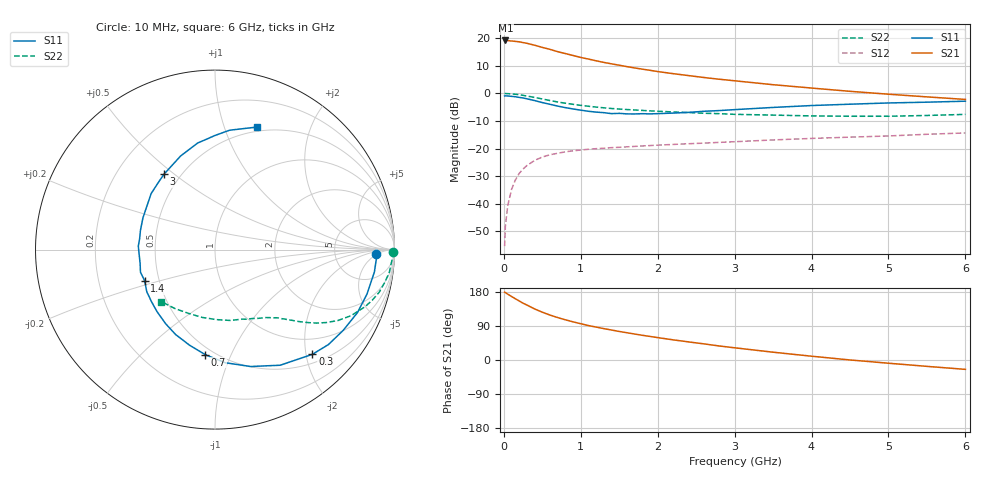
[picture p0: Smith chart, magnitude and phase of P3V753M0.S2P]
! SIEMENS Small Signal Semiconductors
! BFP181
! Si NPN RF Bipolar Junction Transistor in SOT143
! VCE = 0.75 V  IC = 3 mA
! Common Emitter S-Parameters:  March  1996
# GHz  S  MA  R  50
!  f  S11  S21  S12  S22
! GHz  MAG  ANG  MAG  ANG  MAG  ANG  MAG  ANG
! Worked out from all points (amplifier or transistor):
!   36 points, 10 MHz to 6 GHz, reference 50 ohm
!   highest |S21| = 19.2 dB at 20 MHz (marker M1)
!   |S21| within 3 dB of that: start of sweep to 567.7 MHz
!   unconditionally stable (mu >= 1): 1.812 GHz to end of sweep
!   at 250 MHz: K = 0.18, MSG = 22.9 dB, |S12| = -27.4 dB
!   at 1.4 GHz: K = 0.85, MSG = 15.2 dB, |S12| = -19.7 dB
!   at 6 GHz: K = 1.20, MAG = 3.3 dB, |S12| = -14.3 dB
!   S11 on the Smith chart (normalised r, x): 10 MHz: 17, -4; 300 MHz: 0.66, -2.12; 700 MHz: 0.45, -0.80; 1.4 GHz: 0.41, -0.18; 3 GHz: 0.41, +0.46; 6 GHz: 0.46, +1.29
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0.01  0.8949 -1.6  9.071 179.0  0.0017 85.1  0.9908 -0.7
0.02  0.9002 -3.5  9.09 178.1  0.0039 86.3  0.9935 -1.6
0.05  0.8968 -8.0  9.04 173.8  0.0091 86.5  0.9865 -3.9
0.1  0.8823 -16.3  8.885 167.7  0.0181 79.2  0.979 -7.6
0.15  0.8678 -23.9  8.75 161.6  0.0269 75.8  0.9623 -11.1
0.2  0.8442 -32.2  8.582 155.7  0.0354 72.0  0.945 -14.6
0.25  0.8243 -39.9  8.312 149.9  0.0425 67.4  0.9198 -17.9
0.3  0.7967 -47.1  8.076 145.1  0.0492 63.7  0.895 -20.8
0.4  0.7395 -60.6  7.447 134.8  0.0608 57.2  0.8428 -25.9
0.5  0.6808 -73.1  6.798 126.1  0.0702 51.1  0.7904 -30.0
0.6  0.6326 -84.9  6.269 118.6  0.0771 46.6  0.7405 -33.3
0.7  0.5877 -95.3  5.689 112.0  0.0821 42.9  0.6981 -35.9
0.9  0.5215 -114.9  4.853 100.7  0.091 37.2  0.633 -39.6
1.1  0.473 -133.1  4.183 90.8  0.0969 33.6  0.5833 -42.5
1.4  0.4289 -156.0  3.426 79.1  0.1038 29.7  0.5318 -46.3
1.8  0.4277 177.4  2.745 65.2  0.1114 27.0  0.4904 -50.7
2.2  0.4388 156.2  2.275 53.2  0.1185 24.7  0.4605 -55.9
3  0.5069 124.2  1.689 32.2  0.1328 21.2  0.4167 -68.4
3.5  0.5555 110.2  1.435 20.6  0.1431 19.2  0.4035 -78.0
4.5  0.6358 90.0  1.088 0.1  0.1608 14.0  0.3845 -100.8
5.5  0.6919 76.9  0.863 -16.8  0.1812 9.9  0.3973 -124.2
6  0.7209 71.2  0.776 -24.7  0.1917 6.8  0.4159 -135.8
